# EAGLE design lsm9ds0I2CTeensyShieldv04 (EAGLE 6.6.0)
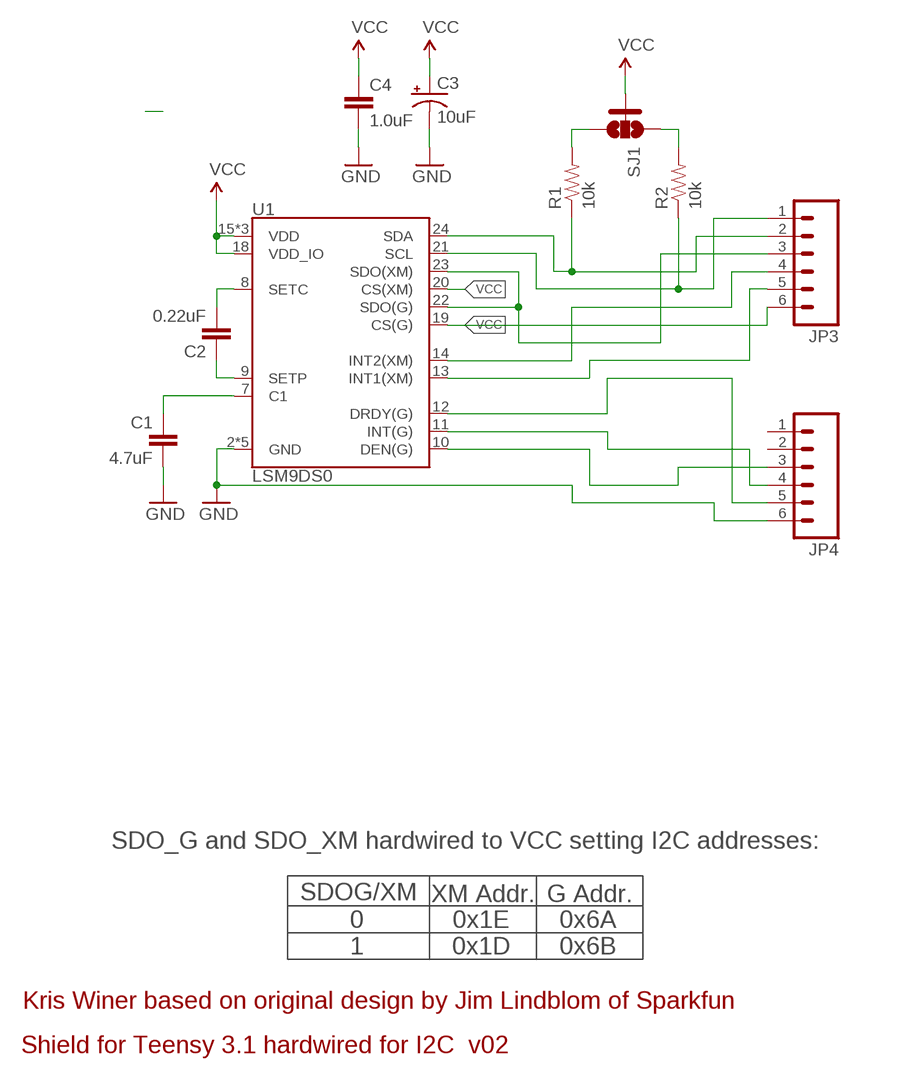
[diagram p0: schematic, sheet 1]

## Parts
C1  4.7uF  4.7UF-6.3V-10%(0603)0603  [0603-CAP]
C2  0.22uF  0.22UF-25V-10%(0603)  [0603-CAP]
C3  10uF  10UF-16V-10%(TANT)  [EIA3216]
C4  1.0uF  1.0UF-16V-10%(0603)  [0603-CAP]
JP3  M06NO_SILK  [1X06_NO_SILK]
JP4  M06NO_SILK  [1X06_NO_SILK]
R1  10k  10K-1%RES-00824  [0603-RES]
R2  10k  10K-1%RES-00824  [0603-RES]
SJ1  SOLDERJUMPER_2WAYS  [SJ_3]
U1  LSM9DS0  [LGA-24]

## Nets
GND: C1.2 C3.C(-) C4.2 JP4.6 U1.2(GND) U1.3(GND) U1.4(GND) U1.5(GND) U1.6(GND)
INT1_XM: JP3.5 U1.13(INT1(XM))
N$1: C2.1 U1.9(SETP)
N$2: C2.2 U1.8(SETC)
N$3: C1.1 U1.7(C1)
N$4: JP4.4 U1.11(INT(G))
N$6: JP4.3 U1.10(DEN(G))
N$7: JP3.4 U1.14(INT2(XM))
N$8: JP4.5 U1.12(DRDY(G))
N$9: R1.2 SJ1.3
N$10: R2.2 SJ1.1
SCL: JP3.2 R1.1 U1.24(SDA)
SDA: JP3.1 R2.1 U1.21(SCL)
SDO: JP3.3 U1.22(SDO(G)) U1.23(SDO(XM))
VCC: C3.A(+) C4.1 JP3.6 SJ1.2 U1.15(VDD) U1.16(VDD) U1.17(VDD) U1.18(VDD_IO) U1.19(CS(G)) U1.20(CS(XM))
Unconnected: JP4.1 JP4.2

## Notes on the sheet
- SDO_G and SDO_XM hardwired to VCC setting I2C addresses:
- SDOG/XM | XM Addr. | G Addr.
- 0
  1
- 0x1E
  0x1D
- 0x6A
  0x6B
- Kris Winer based on original design by Jim Lindblom of Sparkfun
- Shield for Teensy 3.1 hardwired for I2C  v02

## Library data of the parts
C1 = SparkFun-Capacitors:4.7UF-6.3V-10%(0603): CAP-08280; PROD_ID: CAP-08280
C2 = SparkFun-Capacitors:0.22UF-25V-10%(0603): CAP-07822; PROD_ID: CAP-07822
C3 = SparkFun-Capacitors:10UF-16V-10%(TANT): CAP-00811; PROD_ID: CAP-00811
C4 = SparkFun-Capacitors:1.0UF-16V-10%(0603): CAP-00868; PROD_ID: CAP-00868
JP3 JP4 = SparkFun-Connectors:M06: Header 6 Standard 6-pin 0.1" header. Use with straight break away headers (SKU : PRT-00116), right angle break away headers (PRT-00553), swiss pins (PRT-00743), machine pins (PRT-00117), and female headers (PRT-00115). Molex polarized connector foot print use with SKU : PRT-08094 with associated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
R1 R2 = SparkFun-Resistors:10K-1%: 10k-ohm SMT; PROD_ID: RES-00824
SJ1 = SparkFun-Passives:SOLDERJUMPER_2WAY: Solder Jumper 2 way solder jumper
U1 = SparkFun-DigitalIC:LSM9DS0: LSM9DS0 3D Accelerometer, 3D Gyroscope, 3D Magnetomter Features: 3 acceleration channels, 3 angular rate channels, 3 magnetic field channels ±2/±4/±6/±8/±16 g linear acceleration full scale ±2/±4/±8/±12 gauss magnetic full scale ±245/±500/±2000 dps angular rate full scale 16-bit data output SPI /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

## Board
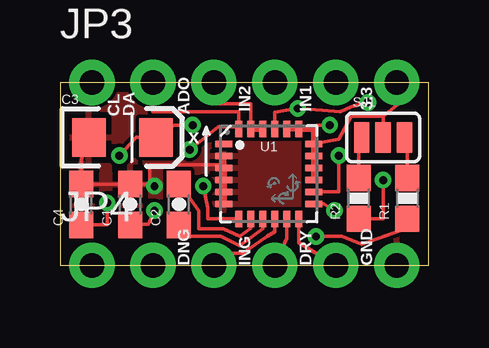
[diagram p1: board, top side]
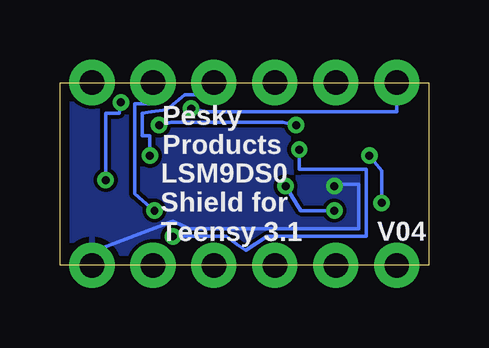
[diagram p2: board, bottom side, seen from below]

Size 15.37 x 7.62 mm. Coordinates in mm from the lower left corner, seen from the top.
Outline: 15.37,0 15.37,7.62 0,7.62 0,0 15.37,0
Copper layers (1*16): Top 0.0356mm / dielectric 1.5011mm / Bottom 0.0356mm
Design rules "OSHPark *": minimum track width 6mil, minimum drill 13mil, track to track 6mil, track to pad 6mil, pad to pad 6mil, via to via 6mil, smd to smd 6mil, copper to edge 15mil, drill to drill 6mil, minimum pad ring 7mil, minimum via ring 7mil, stop-mask expansion 3mil, vias tented up to drill 20mil, thermal gap 10mil

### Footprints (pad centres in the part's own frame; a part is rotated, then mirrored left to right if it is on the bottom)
0603-CAP = smd 1.1 x 1: 1 -0.85,0; 2 0.85,0
EIA3216 = smd 1.4 x 1.6: A 1.4,0; C -1.4,0
1X06_NO_SILK = drill 1.016 pad 1.88: 1 0,0; 2 2.54,0; 3 5.08,0; 4 7.62,0; 5 10.16,0; 6 12.7,0
0603-RES = smd 1.1 x 1: 1 -0.85,0; 2 0.85,0
SJ_3 = smd 0.635 x 1.27: 1 -0.889,0; 2 0,0; 3 0.889,0
LGA-24 = smd 0.7 x 0.29: 1 -1.875,1.25; 2 -1.875,0.75; 3 -1.875,0.25; 4 -1.875,-0.25; 5 -1.875,-0.75; 6 -1.875,-1.25; 13 1.875,-1.25; 14 1.875,-0.75; 15 1.875,-0.25; 16 1.875,0.25; 17 1.875,0.75; 18 1.875,1.25 | smd 0.29 x 0.7: 7 -1.25,-1.875; 8 -0.75,-1.875; 9 -0.25,-1.875; 10 0.25,-1.875; 11 0.75,-1.875; 12 1.25,-1.875; 19 1.25,1.875; 20 0.75,1.875; 21 0.25,1.875; 22 -0.25,1.875; 23 -0.75,1.875; 24 -1.25,1.875

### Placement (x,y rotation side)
C1  2.92,2.54 90 top
C2  4.95,2.54 90 top
C3  2.6,5.33 0 top
C4  0.89,2.54 90 top
JP3  1.33,7.62 0 top
JP4  1.33,0 0 top
R1  14.48,2.79 90 top
R2  12.45,2.79 90 top
SJ1  13.46,5.33 0 top
U1  8.7,3.81 0 top

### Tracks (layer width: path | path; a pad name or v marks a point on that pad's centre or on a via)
GND  (via drill 0.33)
  Top 0.152: C3.C 0.89,4.4 C4.2 C1.2 3.75,3.39 | 3.75,3.39 3.75,4.19 6.82,4.19 | v3.94,3.3 3.81,3.37 3.75,3.39
  Top 0.254: U1.6 U1.5 U1.4 U1.3 6.82,4.19 U1.2
  Bottom 0.152: JP4.6 14.03,0.57 10.67,1.84 9.97,1.52 2.92,1.52 C1.2 3.75,3.39 v3.94,3.3
  pour Top: 0,7.62 0,0 15.37,0 15.37,7.62
  pour Bottom: 0,7.62 0,0 15.37,0 15.37,7.62
INT1_XM  (via drill 0.33)
  Top 0.152: v11.43,2.29 10.99,2.56 U1.13
  Bottom 0.152: v11.43,2.29 12.26,2.98 12.26,6.73 11.49,6.73 JP3.5
N$1
  Top 0.152: U1.9 8.45,1.53 7.49,0.83 6.71,1.21 5.02,1.21 C2.1
N$2
  Top 0.152: U1.8 7.95,1.55 7.49,1.21 6.79,1.52 5.78,1.52 5.78,2.29 5.02,3.37
  Top 0.254: 5.02,3.37 C2.2
N$3  (via drill 0.33)
  Top 0.152: U1.7 6.16,1.94 6.16,2.41 v5.97,3.3 | v3.94,2.29 3.75,1.84 3.68,1.71 2.92,1.71
  Top 0.254: 2.92,1.71 C1.1
  Bottom 0.152: v5.97,3.3 5.33,2.29 v3.94,2.29
N$4
  Top 0.152: JP4.4 9.45,1.14 U1.11
N$6
  Top 0.152: U1.10 8.95,1.4 8.64,1.21 7.62,0.51 6.41,0.51 JP4.3
N$7  (via drill 0.33)
  Top 0.152: U1.14 11.62,3.06 v11.62,4.57
  Bottom 0.152: v11.62,4.57 11.62,5.4 11.94,5.4 11.94,6.35 11.56,6.41 10.92,6.48 10.16,7.11 8.95,7.11 JP3.4
N$8
  Top 0.152: JP4.5 9.95,0.95 U1.12
N$9
  Top 0.152: SJ1.3 14.48,5.14 R1.2
N$10
  Top 0.152: SJ1.1 12.45,5.02 R2.2
SCL  (via drill 0.33)
  Top 0.152: JP3.2 3.87,6.41 7.45,6.41 U1.24 7.45,5.78 6.6,5.78 v5.4,4.83 | v10.67,1.21 11.75,1.21 12.57,0.89 14.22,1.46 R1.1
  Top 0.254: 7.45,5.65 U1.24
  Bottom 0.152: v10.67,1.21 8.45,1.21 8,0.89 7.62,0.64 6.73,1.21 2.6,1.21 2.6,4 5.4,4 v5.4,4.83
SDA  (via drill 0.33)
  Top 0.152: U1.21 8.95,6.39 v9.91,6.54 11.68,6.41 12.13,6.6 v12.83,6.79 | R2.1 13.46,1.94 v13.46,3.56
  Bottom 0.152: JP3.1 1.33,6.41 9.27,6.41 v9.91,6.54 | v13.46,3.56 13.46,6.35 12.89,6.35 v12.83,6.79
SDO
  Top 0.152: U1.23 7.94,6.01 7.94,6.73 6.41,6.73 JP3.3
  Top 0.254: U1.23 U1.22
VCC  (via drill 0.33)
  Top 0.152: JP3.6 14.03,6.67 13.46,6.22 | 13.46,6.22 SJ1.2 | U1.18 11.62,5.25 12.13,6.22 13.46,6.22 | C3.A 4.13,5.33 | C3.A 3.17,5.33 v2.48,4.57 | C3.A 4.76,5.84 v5.52,5.84 | v11.24,5.84 10.7,5.84 10.57,5.68 | C4.1 1.97,1.69 v1.97,2.6
  Top 0.254: U1.15 U1.16 U1.17 U1.18 10.57,5.68 U1.19 U1.20
  Bottom 0.152: v5.52,5.84 6.1,5.97 10.73,5.97 v11.24,5.84 | v1.97,2.6 1.97,3.94 v2.48,4.57

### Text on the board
tPlace: CL | DA | ADO | IN2 | IN1 | 3.3 | x | DNG | ING | DRY | GND
bPlace: Pesky / Products | LSM9DS0 / Shield for / Teensy 3.1 | V04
